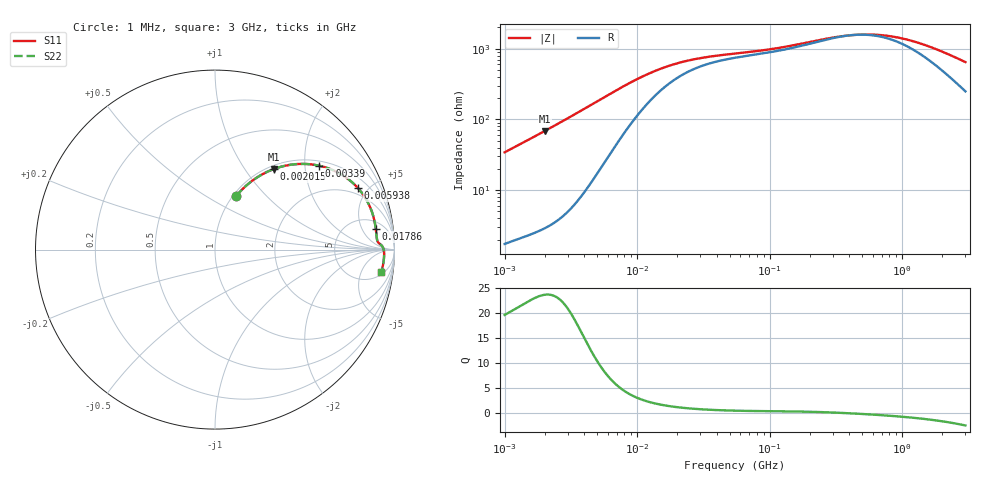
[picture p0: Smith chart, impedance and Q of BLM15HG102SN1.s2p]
! BLM15HG102SN1
# Hz S RI R 50
!Freq.(Hz) S11(Real) S11(Imag) S21(Real) S21(Imag) S12(Real) S12(Imag) S22(Real) S22(Imag)
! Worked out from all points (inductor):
!   401 points, 1 MHz to 3 GHz, reference 50 ohm
!   read as one part in series: L = 5.43 uH near 1.041 MHz
!   highest Q = 23.8 at 2.015 MHz (marker M1), where L = 5.43 uH
!   self-resonance near 428.8 MHz
!   S11 on the Smith chart (normalised r, x): 1 MHz: 1.03, +0.68; 2.015 MHz: 1.06, +1.38; 3.39 MHz: 1.13, +2.37; 5.938 MHz: 1.56, +4.32; 17.86 MHz: 8, +10; 3 GHz: 6, -12
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1000000  0.1169 0.2969  0.8831 -0.2969  0.8831 -0.2969  0.1169 0.2969
1433740  0.2036 0.3806  0.7964 -0.3806  0.7964 -0.3806  0.2036 0.3806
2014875  0.3284 0.449  0.6716 -0.449  0.6716 -0.449  0.3284 0.449
2613693  0.4499 0.476  0.5501 -0.476  0.5501 -0.476  0.4499 0.476
3390478  0.5799 0.4675  0.4201 -0.4675  0.4201 -0.4675  0.5799 0.4675
3823119  0.637 0.4507  0.363 -0.4507  0.363 -0.4507  0.637 0.4507
4764734  0.7284 0.403  0.2716 -0.403  0.2716 -0.403  0.7284 0.403
5938264  0.7967 0.3425  0.2033 -0.3425  0.2033 -0.3425  0.7967 0.3425
8686058  0.8629 0.2396  0.1371 -0.2396  0.1371 -0.2396  0.8629 0.2396
1.461624e7  0.8922 0.1403  0.1078 -0.1403  0.1078 -0.1403  0.8922 0.1403
1.785516e7  0.8959 0.115  0.1041 -0.115  0.1041 -0.115  0.8959 0.115
2.886629e7  0.9003 0.0741  0.0997 -0.0741  0.0997 -0.0741  0.9003 0.0741
5.477226e7  0.905 0.0471  0.095 -0.0471  0.095 -0.0471  0.905 0.0471
1.103592e8  0.9157 0.0341  0.0843 -0.0341  0.0843 -0.0341  0.9157 0.0341
2.094008e8  0.9297 0.0215  0.0703 -0.0215  0.0703 -0.0215  0.9297 0.0215
3.188066e8  0.9368 0.00963  0.0632 -0.00963  0.0632 -0.00963  0.9368 0.00963
4.391493e8  0.9401 -0.000812  0.0599 0.000812  0.0599 0.000812  0.9401 -0.000812
5.929311e8  0.9418 -0.0117  0.0582 0.0117  0.0582 0.0117  0.9418 -0.0117
8.005644e8  0.9424 -0.0241  0.0576 0.0241  0.0576 0.0241  0.9424 -0.0241
1.059487e9  0.9421 -0.0377  0.0579 0.0377  0.0579 0.0377  0.9421 -0.0377
1.430499e9  0.9406 -0.0557  0.0594 0.0557  0.0594 0.0557  0.9406 -0.0557
3e9  0.9271 -0.1247  0.0729 0.1247  0.0729 0.1247  0.9271 -0.1247
